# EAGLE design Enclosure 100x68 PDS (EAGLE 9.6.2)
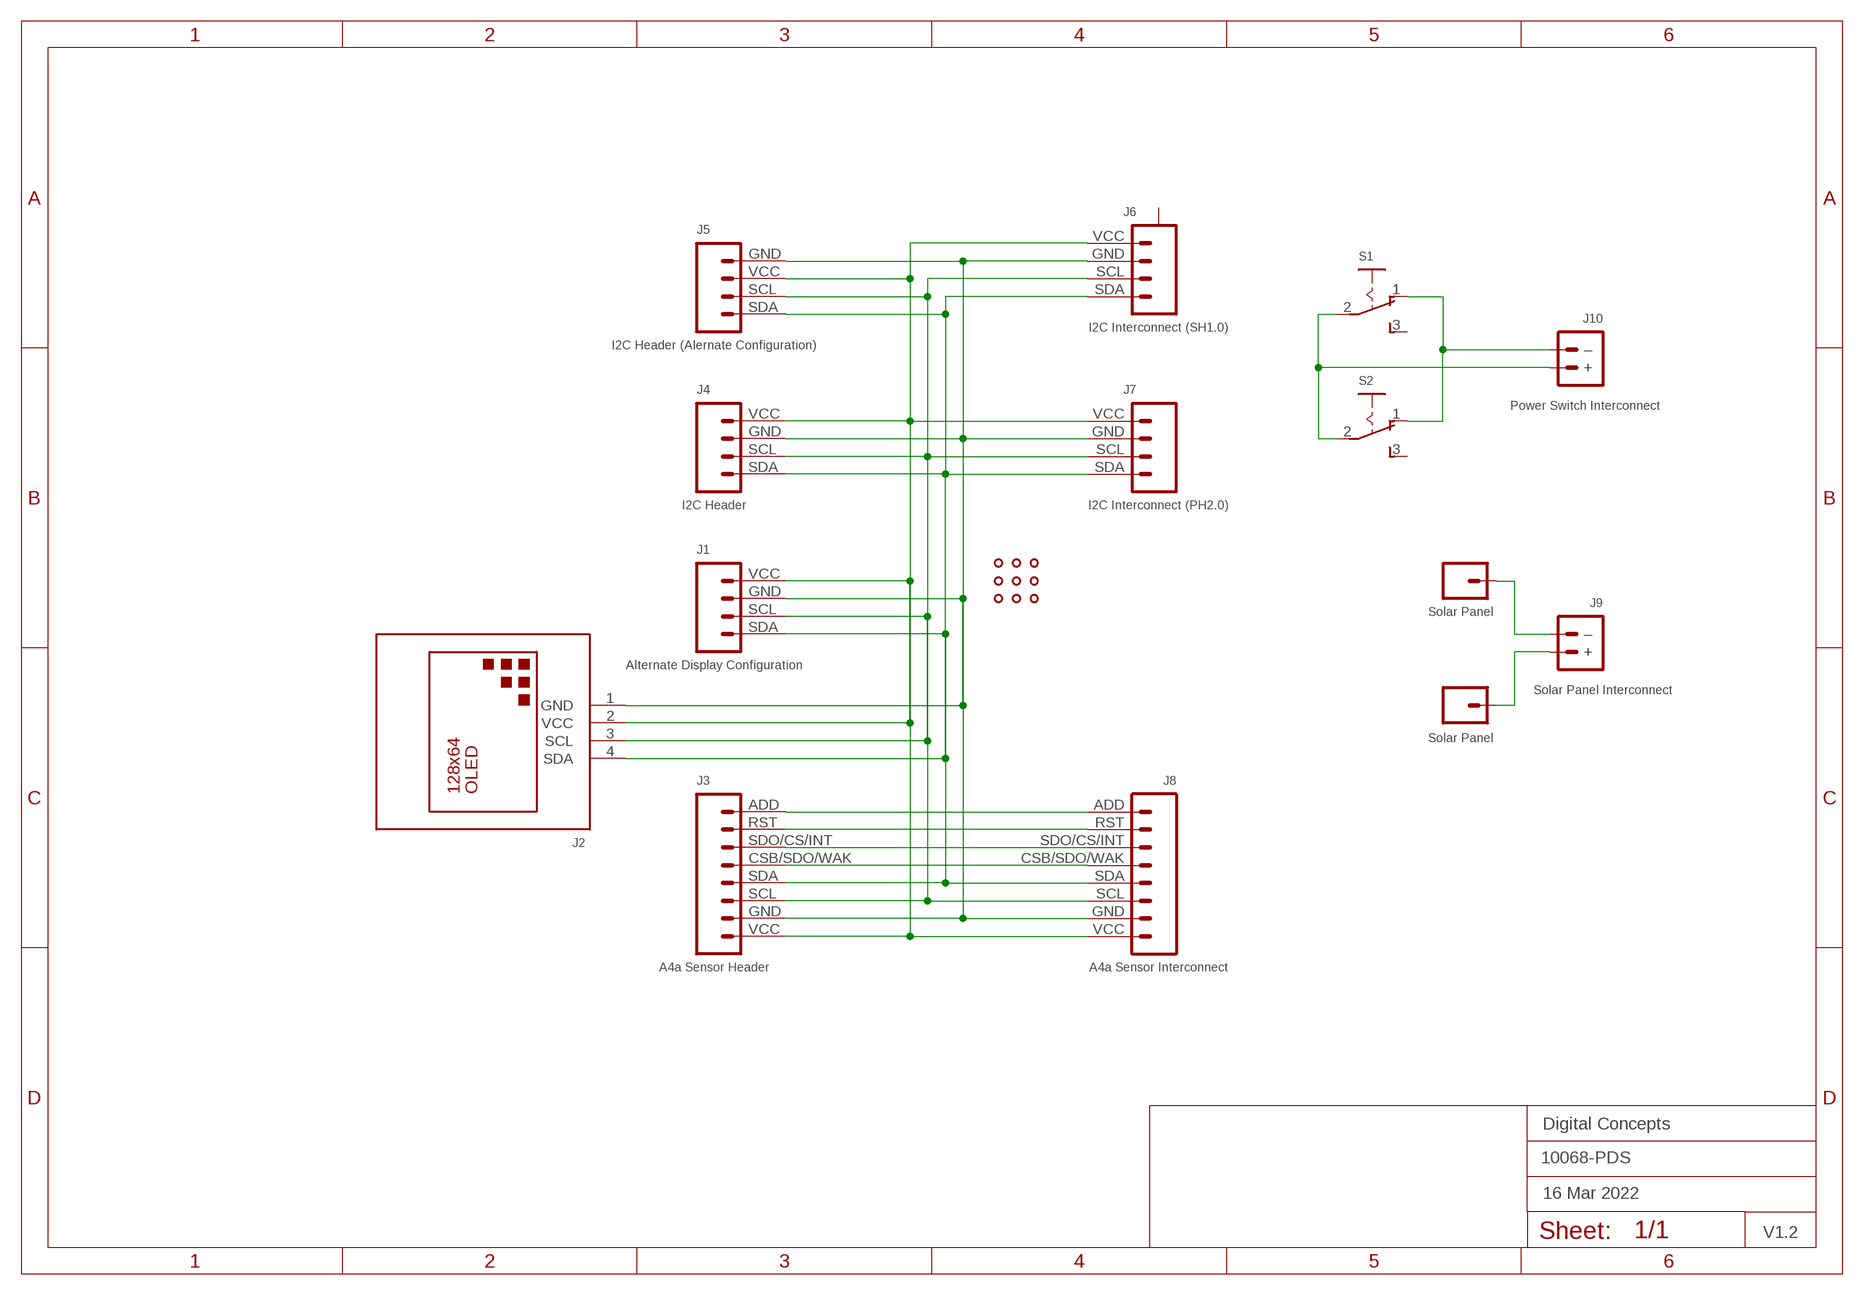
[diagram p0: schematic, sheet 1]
FRAME2 (FRAME-A4L-LOC): DATE: 16 Mar 2022; OWNER: Digital Concepts; TITLE: 10068-PDS; VERSION: V1.2

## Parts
+  Solar Panel  PAD-SMD-GENERIC-SQUARE  [PAD-SMD-GENERIC]
-  Solar Panel  PAD-SMD-GENERIC-SQUARE  [PAD-SMD-GENERIC]
J1  Alternate Display Configuration  HEADER-1X4-I2C  [CONN_04-I2C]
J2  DISPLAY-OLED-128X64-OFFSET-X-I2C  [DISPLAY-OLED-128X64-OFFSET-X-I2C]
J3  A4a Sensor Header  HEADER-1X8-ALF4ALL-SENSOR  [CONN_08-SENSOR]
J4  I2C Header  HEADER-1X4-I2C  [CONN_04-I2C]
J5  I2C Header (Alernate Configuration)  HEADER-1X4-I2C-X  [CONN_04-I2C-X]
J6  I2C Interconnect (SH1.0)  JST-SH1.0-4-I2C-HORIZONTAL  [JST-SH1.0-4-I2C-HORIZONTAL]
J7  I2C Interconnect (PH2.0)  JST-PH2.0-4-I2C-HORIZONTAL  [JST-PH2.0-4-HORIZONTAL]
J8  A4a Sensor Interconnect  HEADER-1X8-ALF4ALL-SENSOR  [CONN_08-SENSOR]
J9  Solar Panel Interconnect  JST-PH2.0-2-HORIZONTALJST-PTH-2  [JST-PH2.0-2-HORIZONTAL]
J10  Power Switch Interconnect  JST-PH2.0-2-HORIZONTALJST-PTH-2  [JST-PH2.0-2-HORIZONTAL]
S1  SWITCH-SLIDE-SPDT  [SWITCH-SPDT-PTH]
S2  SWITCH-SLIDE-SPDT  [SWITCH-SPDT-PTH]
U$1  PROTO-34X22-JST-DS  [PROTO-34X22-JST-DS]

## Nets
GND: J1.GND J2.1(GND) J3.GND J4.GND J5.GND J6.GND J7.GND J8.GND
N$1: J1.SDA J2.4(SDA) J3.SDA J4.SDA J5.SDA J6.SDA J7.SDA J8.SDA
N$2: J1.SCL J2.3(SCL) J3.SCL J4.SCL J5.SCL J6.SCL J7.SCL J8.SCL
N$3: J3.CSB/SDO/WAK J8.CSB/SDO/WAK
N$4: J3.SDO/CS/INT J8.SDO/CS/INT
N$5: J3.RST J8.RST
N$6: J3.ADD J8.ADD
N$7: -.P$1 J9.2(–)
N$8: +.P$1 J9.1(+)
N$10: J10.1(+) S1.2(P) S2.2(P)
N$11: J10.2(–) S1.1(O) S2.1(O)
VCC: J1.VCC J2.2(VCC) J3.VCC J4.VCC J5.VCC J6.VCC J7.VCC J8.VCC
Unconnected: J6.A@1(A) J6.A@4(A) S1.3(S) S2.3(S)

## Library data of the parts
+ - = digitalconcepts:PAD-SMD-GENERIC-SQUARE: SMD Pad—Square
J1 J4 = digitalconcepts:HEADER-1X4-I2C: I2C Interface [Pin 1 Vcc] 4-Pin Header
J2 = digitalconcepts:DISPLAY-OLED-128X64-OFFSET-X-I2C: 128x64 Dot Matrix OLED Module based on SSD1306 chip Offset header variant with I2C interface More details available here: http://www.instructables.com/id/Monochrome-096-i2c-OLED-display-with-arduino-SSD13/ SSD1306 datasheet: https://cdn-shop.adafruit.com/datasheets/SSD1306.pdf Click here to find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
J3 J8 = digitalconcepts:HEADER-1X8-ALF4ALL-SENSOR: IoT Sensors 1x8 Pin Header for 'Sandwich' IoT Sensors
J5 = digitalconcepts:HEADER-1X4-I2C-X: I2C Interface [Pin 1 GND] 4-Pin Header
J6 = digitalconcepts:JST-SH1.0-4-I2C-HORIZONTAL: JST SH1.0 SMD 4P I2C horizontal connector
J7 = digitalconcepts:JST-PH2.0-4-I2C-HORIZONTAL: PH2.0 4P I2C Horizontal Connector
J9 J10 = digitalconcepts:JST-PH2.0-2-HORIZONTAL: PH2.0 2P Right Angle PCB Connector; PROD_ID: CONN-09863; SKU: PRT-09914
S1 S2 = digitalconcepts:SWITCH-SLIDE-SPDT: Mini Sliding Switch SPDT
U$1 = digitalconcepts:PROTO-34X22-JST-DS: 34 x 22 Prototyping board with JST connector points and space for OLED Display, various sensor headers and RJ11 sockets to fit an 100 x 68 enclosure

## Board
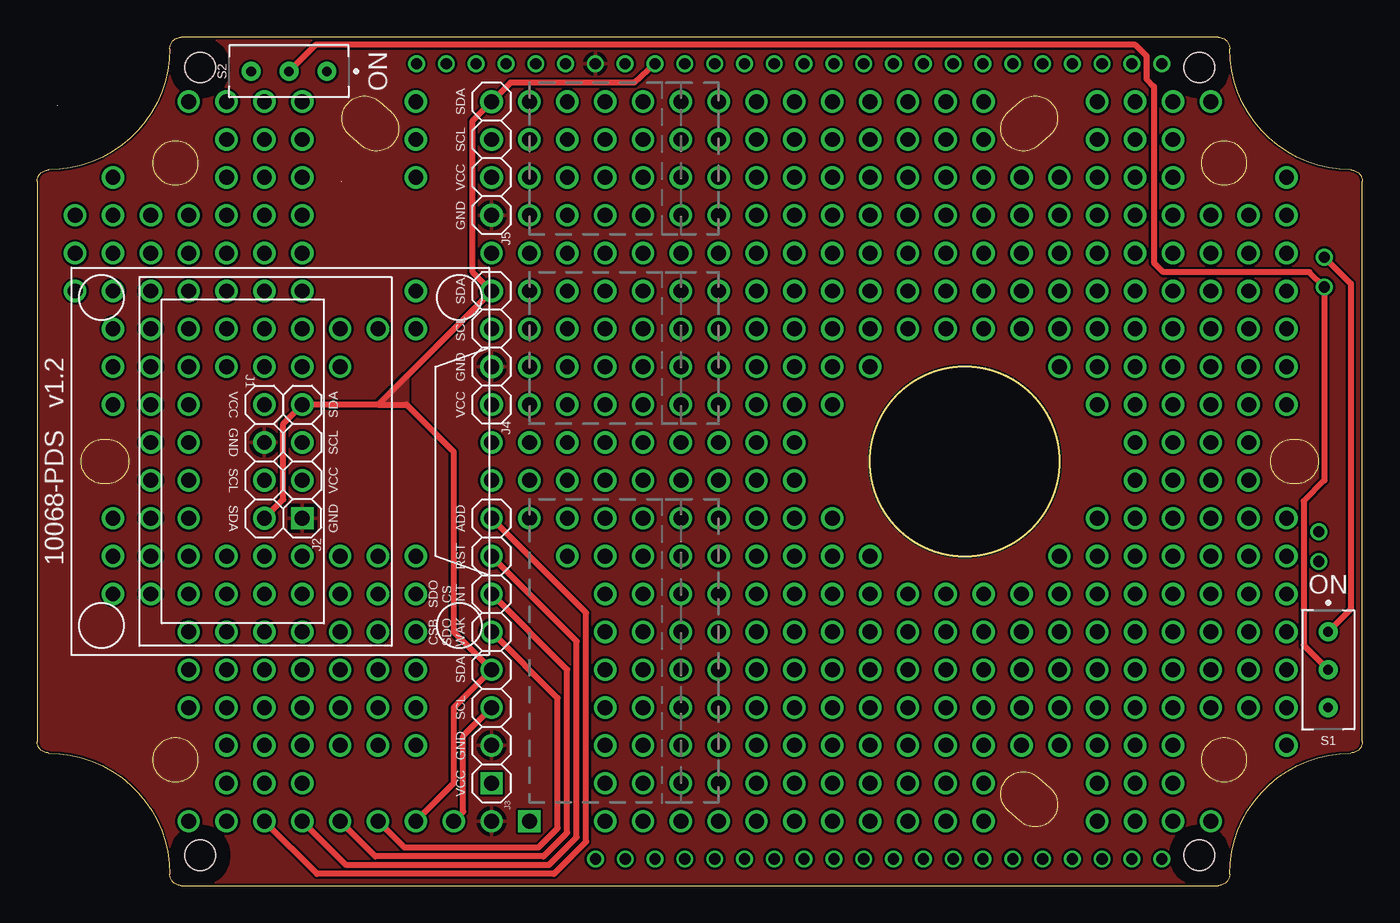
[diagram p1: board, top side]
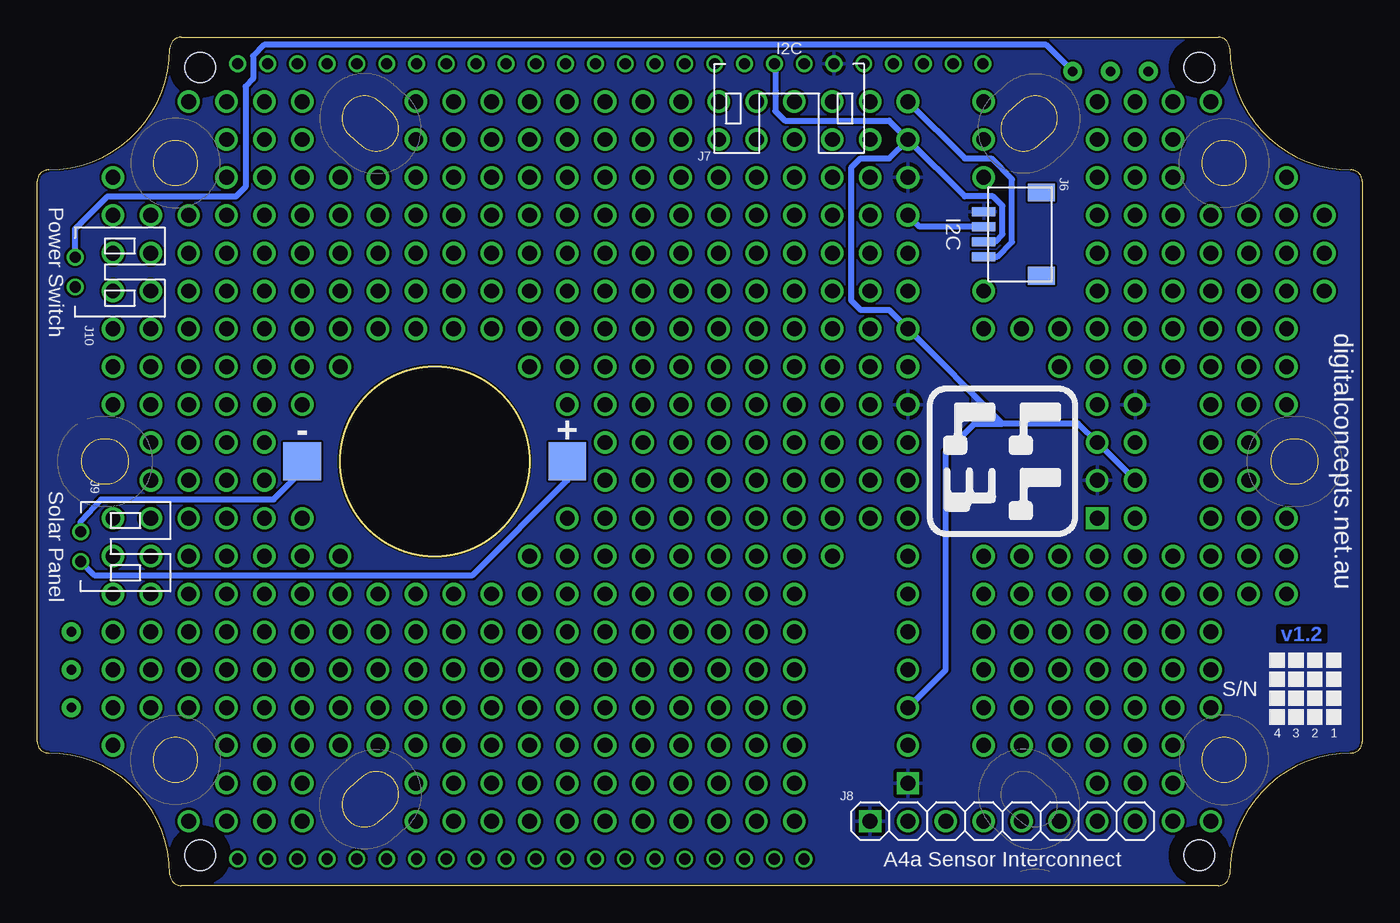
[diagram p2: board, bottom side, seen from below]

Size 88.9 x 56.9 mm. Coordinates in mm from the lower left corner, seen from the top.
Copper layers (1*16): Top 0.035mm / dielectric 1.5mm / Bottom 0.035mm
Design rules "default *": minimum track width 6mil, minimum drill 0.35mm, track to track 6mil, track to pad 6mil, pad to pad 6mil, via to via 6mil, smd to smd 6mil, copper to edge 6mil, drill to drill 6mil, minimum pad ring 1mil, minimum via ring 8mil, stop-mask expansion 4mil, vias tented up to drill 0mil, thermal gap 10mil

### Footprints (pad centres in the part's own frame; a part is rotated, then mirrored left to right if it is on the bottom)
PAD-SMD-GENERIC = smd 2.54 x 2.54: P$1 0,0
CONN_04-I2C = drill 1 pad 1.524: GND 5.08,0; SCL 2.54,0; SDA 0,0; VCC 7.62,0
DISPLAY-OLED-128X64-OFFSET-X-I2C = drill 1 square: 1 -3.81,0 | drill 1: 2 -1.27,0; 3 1.27,0; 4 3.81,0
CONN_08-SENSOR = drill 1: ADD 17.78,0; CSB/SDO/WAK 10.16,0; GND 2.54,0; RST 15.24,0; SCL 5.08,0; SDA 7.62,0; SDO/CS/INT 12.7,0 | drill 1 square: VCC 0,0
CONN_04-I2C-X = drill 1 pad 1.524: GND 7.62,0; SCL 2.54,0; SDA 0,0; VCC 5.08,0
JST-SH1.0-4-I2C-HORIZONTAL = smd 1.2 x 1.8: A@1 -2.8,-3.875; A@4 2.8,-3.875 | smd 0.6 x 1.55: GND 0.5,0; SCL -0.5,0; SDA -1.5,0; VCC 1.5,0
JST-PH2.0-4-HORIZONTAL = drill 0.75: GND -1,0; SCL 1,0; SDA 3,0; VCC -3,0
JST-PH2.0-2-HORIZONTAL = drill 0.75: 1 1,0; 2 -1,0
SWITCH-SPDT-PTH = drill 0.65 pad 1.27: 1 -2.54,0; 2 0,0; 3 2.54,0
PROTO-34X22-JST-DS = drill 1: P01-16 -41.91,11.43; P01-17 -41.91,13.97; P01-18 -41.91,16.51; P02-08 -39.37,-8.89; P02-09 -39.37,-6.35; P02-10 -39.37,-3.81; P02-13 -39.37,3.81; P02-14 -39.37,6.35; P02-15 -39.37,8.89; P02-16 -39.37,11.43; P02-17 -39.37,13.97; P02-18 -39.37,16.51; P02-19 -39.37,19.05; P03-08 -36.83,-8.89; P03-09 -36.83,-6.35; P03-10 -36.83,-3.81; P03-11 -36.83,-1.27; P03-12 -36.83,1.27; P03-13 -36.83,3.81; P03-14 -36.83,6.35; P03-15 -36.83,8.89; P03-16 -36.83,11.43; P03-17 -36.83,13.97; P03-18 -36.83,16.51; P04-02 -34.29,-24.13; P04-05 -34.29,-16.51; P04-06 -34.29,-13.97; P04-07 -34.29,-11.43; P04-08 -34.29,-8.89; P04-09 -34.29,-6.35; P04-10 -34.29,-3.81; P04-11 -34.29,-1.27; P04-12 -34.29,1.27; P04-13 -34.29,3.81; P04-14 -34.29,6.35; P04-15 -34.29,8.89; P04-16 -34.29,11.43; P04-17 -34.29,13.97; P04-18 -34.29,16.51; P04-21 -34.29,24.13; P05-02 -31.75,-24.13; P05-03 -31.75,-21.59; P05-04 -31.75,-19.05; P05-05 -31.75,-16.51; P05-06 -31.75,-13.97; P05-07 -31.75,-11.43; P05-08 -31.75,-8.89; P05-09 -31.75,-6.35; P05-14 -31.75,6.35; P05-15 -31.75,8.89; P05-16 -31.75,11.43; P05-17 -31.75,13.97; P05-18 -31.75,16.51; P05-19 -31.75,19.05; P05-20 -31.75,21.59; P05-21 -31.75,24.13; P06-03 -29.21,-21.59; P06-04 -29.21,-19.05; P06-05 -29.21,-16.51; P06-06 -29.21,-13.97; P06-07 -29.21,-11.43; P06-08 -29.21,-8.89; P06-09 -29.21,-6.35; P06-14 -29.21,6.35; P06-15 -29.21,8.89; P06-16 -29.21,11.43; P06-17 -29.21,13.97; P06-18 -29.21,16.51; P06-19 -29.21,19.05; P06-20 -29.21,21.59; P06-21 -29.21,24.13; P07-03 -26.67,-21.59; P07-04 -26.67,-19.05; P07-05 -26.67,-16.51; P07-06 -26.67,-13.97; P07-07 -26.67,-11.43; P07-08 -26.67,-8.89; P07-09 -26.67,-6.35; P07-14 -26.67,6.35; P07-15 -26.67,8.89; P07-16 -26.67,11.43; P07-17 -26.67,13.97; P07-18 -26.67,16.51; P07-19 -26.67,19.05; P07-20 -26.67,21.59; P07-21 -26.67,24.13; P08-04 -24.13,-19.05; P08-05 -24.13,-16.51; P08-06 -24.13,-13.97; P08-07 -24.13,-11.43; P08-08 -24.13,-8.89; P08-09 -24.13,-6.35; P08-14 -24.13,6.35; P08-15 -24.13,8.89; P09-04 -21.59,-19.05; P09-05 -21.59,-16.51; P09-06 -21.59,-13.97; P09-07 -21.59,-11.43; P09-08 -21.59,-8.89; P09-09 -21.59,-6.35; P09-15 -21.59,8.89; P10-04 -19.05,-19.05; P10-05 -19.05,-16.51; P10-06 -19.05,-13.97; P10-07 -19.05,-11.43; P10-08 -19.05,-8.89; P10-09 -19.05,-6.35; P10-15 -19.05,8.89; P10-16 -19.05,11.43; P10-19 -19.05,19.05; P10-20 -19.05,21.59; P10-21 -19.05,24.13; P12-11 -13.97,-1.27; P12-12 -13.97,1.27; P12-17 -13.97,13.97; P13-10 -11.43,-3.81; P13-11 -11.43,-1.27; P13-12 -11.43,1.27; P13-13 -11.43,3.81; P13-14 -11.43,6.35; P13-15 -11.43,8.89; P13-16 -11.43,11.43; P13-17 -11.43,13.97; P13-18 -11.43,16.51; P13-19 -11.43,19.05; P13-20 -11.43,21.59; P13-21 -11.43,24.13; P14-09 -8.89,-6.35; P14-10 -8.89,-3.81; P14-11 -8.89,-1.27; P14-12 -8.89,1.27; P14-13 -8.89,3.81; P14-14 -8.89,6.35; P14-15 -8.89,8.89; P14-16 -8.89,11.43; P14-17 -8.89,13.97; P14-18 -8.89,16.51; P14-19 -8.89,19.05; P14-20 -8.89,21.59; P14-21 -8.89,24.13; P15-02 -6.35,-24.13; P15-03 -6.35,-21.59; P15-04 -6.35,-19.05; P15-05 -6.35,-16.51; P15-06 -6.35,-13.97; P15-07 -6.35,-11.43; P15-08 -6.35,-8.89; P15-09 -6.35,-6.35; P15-10 -6.35,-3.81; P15-11 -6.35,-1.27; P15-12 -6.35,1.27; P15-13 -6.35,3.81; P15-14 -6.35,6.35; P15-15 -6.35,8.89; P15-16 -6.35,11.43; P15-17 -6.35,13.97; P15-18 -6.35,16.51; P15-19 -6.35,19.05; P15-20 -6.35,21.59; P15-21 -6.35,24.13; P16-02 -3.81,-24.13; P16-03 -3.81,-21.59; P16-04 -3.81,-19.05; P16-05 -3.81,-16.51; P16-06 -3.81,-13.97; P16-07 -3.81,-11.43; P16-08 -3.81,-8.89; P16-09 -3.81,-6.35; P16-10 -3.81,-3.81; P16-11 -3.81,-1.27; P16-12 -3.81,1.27; P16-13 -3.81,3.81; P16-14 -3.81,6.35; P16-15 -3.81,8.89; P16-16 -3.81,11.43; P16-17 -3.81,13.97; P16-18 -3.81,16.51; P16-19 -3.81,19.05; P16-20 -3.81,21.59; P16-21 -3.81,24.13; P17-02 -1.27,-24.13; P17-03 -1.27,-21.59; P17-04 -1.27,-19.05; P17-05 -1.27,-16.51; P17-06 -1.27,-13.97; P17-07 -1.27,-11.43; P17-08 -1.27,-8.89; P17-09 -1.27,-6.35; P17-10 -1.27,-3.81; P17-11 -1.27,-1.27; P17-12 -1.27,1.27; P17-13 -1.27,3.81; P17-14 -1.27,6.35; P17-15 -1.27,8.89; P17-16 -1.27,11.43; P17-17 -1.27,13.97; P17-18 -1.27,16.51; P17-19 -1.27,19.05; P17-20 -1.27,21.59; P17-21 -1.27,24.13; P18-02 1.27,-24.13; P18-03 1.27,-21.59; P18-04 1.27,-19.05; P18-05 1.27,-16.51; P18-06 1.27,-13.97; P18-07 1.27,-11.43; P18-08 1.27,-8.89; P18-09 1.27,-6.35; P18-10 1.27,-3.81; P18-11 1.27,-1.27; P18-12 1.27,1.27; P18-13 1.27,3.81; P18-14 1.27,6.35; P18-15 1.27,8.89; P18-16 1.27,11.43; P18-17 1.27,13.97; P18-18 1.27,16.51; P18-19 1.27,19.05; P18-20 1.27,21.59; P18-21 1.27,24.13; P19-02 3.81,-24.13; P19-03 3.81,-21.59; P19-04 3.81,-19.05; P19-05 3.81,-16.51; P19-06 3.81,-13.97; P19-07 3.81,-11.43; P19-08 3.81,-8.89; P19-09 3.81,-6.35; P19-10 3.81,-3.81; P19-11 3.81,-1.27; P19-12 3.81,1.27; P19-13 3.81,3.81; P19-14 3.81,6.35; P19-15 3.81,8.89; P19-16 3.81,11.43; P19-17 3.81,13.97; P19-18 3.81,16.51; P19-19 3.81,19.05; P19-20 3.81,21.59; P19-21 3.81,24.13; P20-02 6.35,-24.13; P20-03 6.35,-21.59; P20-04 6.35,-19.05; P20-05 6.35,-16.51; P20-06 6.35,-13.97; P20-07 6.35,-11.43; P20-08 6.35,-8.89; P20-09 6.35,-6.35; P20-10 6.35,-3.81; P20-11 6.35,-1.27; P20-12 6.35,1.27; P20-13 6.35,3.81; P20-14 6.35,6.35; P20-15 6.35,8.89; P20-16 6.35,11.43; P20-17 6.35,13.97; P20-18 6.35,16.51; P20-19 6.35,19.05; P20-20 6.35,21.59; P20-21 6.35,24.13; P21-02 8.89,-24.13; P21-03 8.89,-21.59; P21-04 8.89,-19.05; P21-05 8.89,-16.51; P21-06 8.89,-13.97; P21-07 8.89,-11.43; P21-08 8.89,-8.89; P21-09 8.89,-6.35; P21-10 8.89,-3.81; P21-13 8.89,3.81; P21-14 8.89,6.35; P21-15 8.89,8.89; P21-16 8.89,11.43; P21-17 8.89,13.97; P21-18 8.89,16.51; P21-19 8.89,19.05; P21-20 8.89,21.59; P21-21 8.89,24.13; P22-02 11.43,-24.13; P22-03 11.43,-21.59; P22-04 11.43,-19.05; P22-05 11.43,-16.51; P22-06 11.43,-13.97; P22-07 11.43,-11.43; P22-08 11.43,-8.89; P22-09 11.43,-6.35; P22-14 11.43,6.35; P22-15 11.43,8.89; P22-16 11.43,11.43; P22-17 11.43,13.97; P22-18 11.43,16.51; P22-19 11.43,19.05; P22-20 11.43,21.59; P22-21 11.43,24.13; P23-02 13.97,-24.13; P23-03 13.97,-21.59; P23-04 13.97,-19.05; P23-05 13.97,-16.51; P23-06 13.97,-13.97; P23-07 13.97,-11.43; P23-08 13.97,-8.89; P23-15 13.97,8.89; P23-16 13.97,11.43; P23-17 13.97,13.97; P23-18 13.97,16.51; P23-19 13.97,19.05; P23-20 13.97,21.59; P23-21 13.97,24.13; P24-02 16.51,-24.13; P24-03 16.51,-21.59; P24-04 16.51,-19.05; P24-05 16.51,-16.51; P24-06 16.51,-13.97; P24-07 16.51,-11.43; P24-08 16.51,-8.89; P24-15 16.51,8.89; P24-16 16.51,11.43; P24-17 16.51,13.97; P24-18 16.51,16.51; P24-19 16.51,19.05; P24-20 16.51,21.59; P24-21 16.51,24.13; P25-02 19.05,-24.13; P25-03 19.05,-21.59; P25-04 19.05,-19.05; P25-05 19.05,-16.51; P25-06 19.05,-13.97; P25-07 19.05,-11.43; P25-08 19.05,-8.89; P25-15 19.05,8.89; P25-16 19.05,11.43; P25-17 19.05,13.97; P25-18 19.05,16.51; P25-19 19.05,19.05; P25-20 19.05,21.59; P25-21 19.05,24.13; P26-04 21.59,-19.05; P26-05 21.59,-16.51; P26-06 21.59,-13.97; P26-07 21.59,-11.43; P26-08 21.59,-8.89; P26-15 21.59,8.89; P26-16 21.59,11.43; P26-17 21.59,13.97; P26-18 21.59,16.51; P26-19 21.59,19.05; P27-04 24.13,-19.05; P27-05 24.13,-16.51; P27-06 24.13,-13.97; P27-07 24.13,-11.43; P27-08 24.13,-8.89; P27-09 24.13,-6.35; P27-14 24.13,6.35; P27-15 24.13,8.89; P27-16 24.13,11.43; P27-17 24.13,13.97; P27-18 24.13,16.51; P27-19 24.13,19.05; P28-02 26.67,-24.13; P28-03 26.67,-21.59; P28-04 26.67,-19.05; P28-05 26.67,-16.51; P28-06 26.67,-13.97; P28-07 26.67,-11.43; P28-08 26.67,-8.89; P28-09 26.67,-6.35; P28-10 26.67,-3.81; P28-13 26.67,3.81; P28-14 26.67,6.35; P28-15 26.67,8.89; P28-16 26.67,11.43; P28-17 26.67,13.97; P28-18 26.67,16.51; P28-19 26.67,19.05; P28-20 26.67,21.59; P28-21 26.67,24.13; P29-02 29.21,-24.13; P29-03 29.21,-21.59; P29-04 29.21,-19.05; P29-05 29.21,-16.51; P29-06 29.21,-13.97; P29-07 29.21,-11.43; P29-08 29.21,-8.89; P29-09 29.21,-6.35; P29-10 29.21,-3.81; P29-11 29.21,-1.27; P29-12 29.21,1.27; P29-13 29.21,3.81; P29-14 29.21,6.35; P29-15 29.21,8.89; P29-16 29.21,11.43; P29-17 29.21,13.97; P29-18 29.21,16.51; P29-19 29.21,19.05; P29-20 29.21,21.59; P29-21 29.21,24.13; P30-02 31.75,-24.13; P30-03 31.75,-21.59; P30-04 31.75,-19.05; P30-05 31.75,-16.51; P30-06 31.75,-13.97; P30-07 31.75,-11.43; P30-08 31.75,-8.89; P30-09 31.75,-6.35; P30-10 31.75,-3.81; P30-11 31.75,-1.27; P30-12 31.75,1.27; P30-13 31.75,3.81; P30-14 31.75,6.35; P30-15 31.75,8.89; P30-16 31.75,11.43; P30-17 31.75,13.97; P30-18 31.75,16.51; P30-19 31.75,19.05; P30-20 31.75,21.59; P30-21 31.75,24.13; P31-02 34.29,-24.13; P31-05 34.29,-16.51; P31-06 34.29,-13.97; P31-07 34.29,-11.43; P31-08 34.29,-8.89; P31-09 34.29,-6.35; P31-10 34.29,-3.81; P31-11 34.29,-1.27; P31-12 34.29,1.27; P31-13 34.29,3.81; P31-14 34.29,6.35; P31-15 34.29,8.89; P31-16 34.29,11.43; P31-17 34.29,13.97; P31-18 34.29,16.51; P31-21 34.29,24.13; P32-05 36.83,-16.51; P32-06 36.83,-13.97; P32-07 36.83,-11.43; P32-08 36.83,-8.89; P32-09 36.83,-6.35; P32-10 36.83,-3.81; P32-11 36.83,-1.27; P32-12 36.83,1.27; P32-13 36.83,3.81; P32-14 36.83,6.35; P32-15 36.83,8.89; P32-16 36.83,11.43; P32-17 36.83,13.97; P32-18 36.83,16.51; P33-04 39.37,-19.05; P33-05 39.37,-16.51; P33-06 39.37,-13.97; P33-07 39.37,-11.43; P33-08 39.37,-8.89; P33-09 39.37,-6.35; P33-10 39.37,-3.81; P33-13 39.37,3.81; P33-14 39.37,6.35; P33-15 39.37,8.89; P33-16 39.37,11.43; P33-17 39.37,13.97; P33-18 39.37,16.51; P33-19 39.37,19.05 | drill 0.75: P12-22 -19,26.67; P13-22 -17,26.67; P14-22 -15,26.67; P15-22 -13,26.67; P16-22 -11,26.67; P18-01 -7,-26.67; P19-01 -5,-26.67; P20-01 -3,-26.67; P21-01 -1,-26.67; P21-22 -1,26.67; P22-01 1,-26.67; P22-22 1,26.67; P23-01 3,-26.67; P23-22 3,26.67; P24-01 5,-26.67; P24-22 5,26.67; P25-01 7,-26.67; P25-22 7,26.67; P26-01 9,-26.67; P26-22 9,26.67; P27-01 11,-26.67; P27-22 11,26.67; P28-01 13,-26.67; P28-22 13,26.67; P29-01 15,-26.67; P29-22 15,26.67; P30-01 17,-26.67; P30-22 17,26.67; P31-01 19,-26.67; P31-22 19,26.67; P32-01 21,-26.67; P32-22 21,26.67; P33-01 23,-26.67; P33-22 23,26.67; P34-01 25,-26.67; P34-22 25,26.67; P35-01 27,-26.67; P35-22 27,26.67; P36-01 29,-26.67; P36-22 29,26.67; P37-01 31,-26.67; P37-22 31,26.67 | hole 2.032: -33.528,26.416; 33.528,26.416; 33.528,-26.416; -33.528,-26.416 | hole 12.7: 17.78,0

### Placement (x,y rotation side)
+  53.34,28.45 0 bottom
-  71.12,28.45 0 bottom
J1  15.24,24.64 90 top
J2  17.78,28.45 90 top
J3  30.48,6.86 90 top
J4  30.48,39.88 270 top
J5  30.48,52.58 270 top
J6  25.4,43.69 90 bottom
J7  38.45,55.12 180 bottom
J8  33.02,4.32 0 bottom
J9  85.98,22.73 270 bottom
J10  86.36,41.15 270 bottom
S1  86.61,14.48 270 top
S2  16.89,54.61 180 top
U$1  44.45,28.45 0 top

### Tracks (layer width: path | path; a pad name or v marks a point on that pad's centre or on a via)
$X0
  cutout Bottom: 10.92,56.9 arc180 10.92,52.83 arc180
$X1
  cutout Bottom: 77.98,56.9 arc180 77.98,52.83 arc180
$X2
  cutout Bottom: 77.98,4.06 arc180 77.98,0 arc180
$X3
  cutout Bottom: 10.92,4.06 arc180 10.92,0 arc180
$X4
  cutout Top: 10.92,56.9 arc180 10.92,52.83 arc180
$X5
  cutout Top: 77.98,56.9 arc180 77.98,52.83 arc180
$X6
  cutout Top: 77.98,4.06 arc180 77.98,0 arc180
$X7
  cutout Top: 10.92,4.06 arc180 10.92,0 arc180
GND
  Bottom 0.406: J6.GND 29.71,44.19 J5.GND
  pour Top (rank 5): -1.27,58.93 90.17,58.93 90.17,-2.03 -1.27,-2.03
N$1
  Top 0.406: J1.SDA 16.51,25.91 16.51,30.99 J2.4 22.86,32.26 | 22.86,32.26 J4.SDA 29.21,41.15 29.21,51.31 J5.SDA 31.75,53.85 40.06,53.85 J7.SDA | 22.86,32.26 24.77,32.26 27.94,29.08 27.94,17.02 J3.SDA 27.94,11.94 27.94,6.86 J8.SDA
  Bottom 0.406: J6.SDA 24.49,42.19 23.5,43.18 23.5,47.37 24.89,48.77 26.67,48.77 J5.SDA
  pour Top: 24.77,32.26 24.77,34.16 22.86,32.26
N$2
  Top 0.406: J8.SCL 28.58,4.95 28.58,10.03 J3.SCL
  Bottom 0.406: J1.SCL J2.3 19.05,30.99 24.13,30.99 | 24.13,30.99 J4.SCL 31.75,38.61 33.66,38.61 34.29,39.24 34.29,48.13 33.66,48.77 31.75,48.77 J5.SCL | J3.SCL 27.94,14.48 27.94,29.08 26.04,30.99 24.13,30.99 | J7.SCL 39.37,54.99 39.37,51.94 38.73,51.31 31.75,51.31 J5.SCL | J6.SCL 24.63,43.19 24.13,43.69 24.13,45.59 24.77,46.23 26.67,46.23 J5.SCL
  pour Bottom: 24.13,30.99 26.04,30.99 26.04,32.89
N$3
  Top 0.406: J3.CSB/SDO/WAK 34.93,12.57 34.93,3.86 33.6,2.54 24.64,2.54 J8.CSB/SDO/WAK
N$4
  Top 0.406: J3.SDO/CS/INT 35.56,14.48 35.56,3.56 33.96,1.96 22.68,1.96 J8.SDO/CS/INT
N$5
  Top 0.406: J3.RST 36.2,16.38 36.2,3.25 34.32,1.37 20.73,1.37 J8.RST
N$6
  Top 0.406: J3.ADD 36.83,18.29 36.83,2.95 34.67,0.79 18.77,0.79 J8.ADD
N$7
  Bottom 0.406: J9.2 85.98,24.43 84.62,25.91 73.03,25.91 71.12,27.81 -.P$1
N$8
  Bottom 0.406: +.P$1 53.34,27.18 59.69,20.83 85.07,20.83 J9.1
N$10
  Top 0.406: S1.2 84.96,16.13 84.96,25.78 86.36,27.18 J10.1 85.36,41.15 75.56,41.15 74.93,41.78 74.93,53.59 74.42,54.1 74.42,55.64 73.66,56.39 18.67,56.39 S2.2
N$11
  Top 0.406: J10.2 88.14,40.37 88.14,18.54 S1.1
  Bottom 0.406: J10.2 86.36,44.05 84.19,46.23 75.56,46.23 74.93,46.86 74.93,53.59 74.42,54.1 74.42,55.63 73.66,56.39 21.21,56.39 S2.1
VCC
  pour Bottom (rank 5): 0,57.66 88.9,57.66 88.9,-0.76 0,-0.76

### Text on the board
Bottom: v1.2
tPlace: ON | SDA | SCL | VCC | GND | SDA | SCL | GND | VCC | VCC | GND | 10068-PDS v1.2 | SCL | SDA | ADD | RST | SDO / CS / INT | ON | CSB / SDO / WAK | SDA | SCL | GND | VCC
bPlace: digitalconcepts.net.au | S/N | 1 | 2 | 3 | 4
bNames: I2C | I2C | Power Switch | Solar Panel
